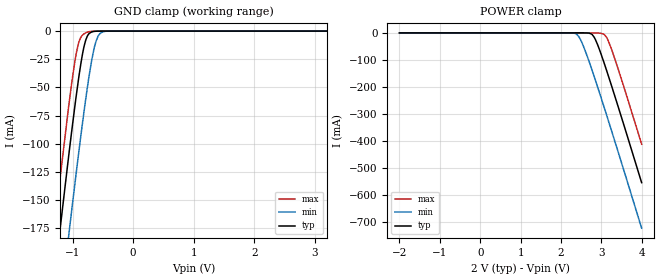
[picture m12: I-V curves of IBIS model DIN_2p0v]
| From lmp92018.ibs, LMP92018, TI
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|   Model
[Model]   DIN_2p0v
Model_type   Input
Vinl = 0.6
Vinh = 1.4
|   typ   min   max
C_comp   0.3672pF   0.3049pF   0.3707pF
[Voltage Range]   2   1.8   2.2
[Temperature Range]   27   125   -40
[Power Clamp Reference]   2   1.8   2.2
[GND Clamp Reference]   0   0   0
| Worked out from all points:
|   GND clamp passes 1 mA (typ) near -0.69 V on its own axis
[GND Clamp]
|   Voltage   I(typ)   I(min)   I(max)
-2V       -557mA     -627.8mA   -512.6mA
-1.55V    -338.6mA   -410.2mA   -293.5mA
-1.262V   -201.6mA   -273.4mA   -156.2mA
-1.226V   -184.7mA   -256.5mA   -139.5mA
-1.058V   -108mA     -178.8mA   -64.21mA
-962mV    -66.66mA   -135.7mA   -26.98mA
-902mV    -42.85mA   -109.4mA   -10.89mA
-782mV    -7.951mA   -60.03mA   -1.575mA
-638mV    -248.3uA   -13.95mA   -53.26uA
-578mV    -53.47uA   -4.443mA   -7.974uA
-494mV    -5.344uA   -538.2uA   0A
3.994V    0A         0A         0A
[POWER Clamp]
|   Voltage   I(typ)   I(min)   I(max)
-2V       0A         0A         0A
2.206V    0A         -48.88uA   0A
2.386V    0A         -5.294mA   0A
2.458V    -1.856uA   -18.71mA   0A
2.53V     -14.69uA   -40.84mA   0A
2.77V     -6.134mA   -139.2mA   -6.055uA
2.902V    -42.85mA   -198.9mA   -301.1uA
3.046V    -102.7mA   -265.8mA   -4.254mA
3.13V     -140.5mA   -305.4mA   -17.29mA
3.238V    -190.3mA   -356.7mA   -55.85mA
3.382V    -258.2mA   -425.6mA   -119.2mA
3.994V    -554.1mA   -722.4mA   -411.9mA
